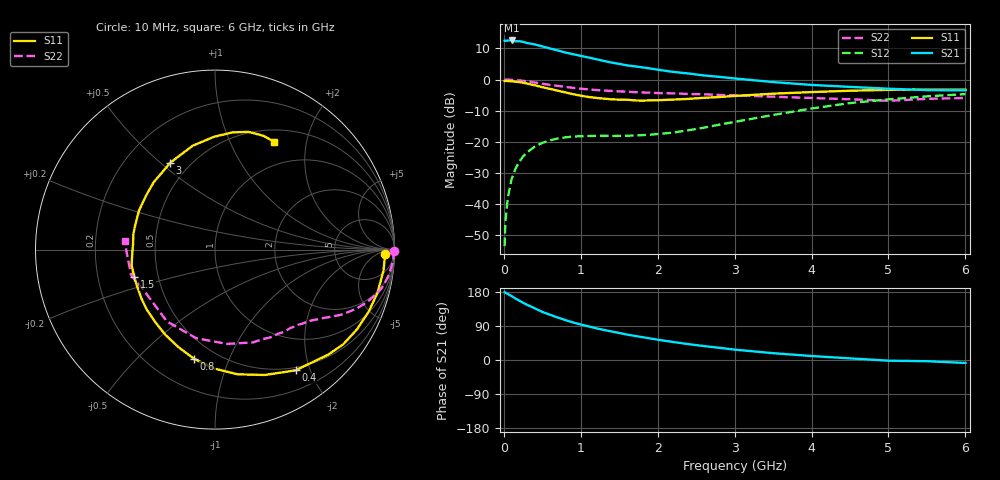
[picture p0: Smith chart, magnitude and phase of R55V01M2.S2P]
! SIEMENS Small Signal Semiconductors
! BFR183
! Si NPN RF Bipolar Junction Transistor in SOT23
! VCE = 5 V  IC = 1.2 mA
! Common Emitter S-Parameters:  May  1996
# GHz  S  MA  R  50
!  f  S11  S21  S12  S22
! GHz  MAG  ANG  MAG  ANG  MAG  ANG  MAG  ANG
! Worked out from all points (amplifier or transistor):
!   36 points, 10 MHz to 6 GHz, reference 50 ohm
!   highest |S21| = 12.5 dB at 100 MHz (marker M1)
!   |S21| within 3 dB of that: start of sweep to 667.1 MHz
!   unconditionally stable (mu >= 1): 1.612 GHz to 2.909 GHz
!   at 250 MHz: K = 0.17, MSG = 18.4 dB, |S12| = -24.7 dB
!   at 1.4 GHz: K = 0.89, MSG = 11.8 dB, |S12| = -18.1 dB
!   at 6 GHz: K = 0.94, MSG = 0.6 dB, |S12| = -4.7 dB
!   S11 on the Smith chart (normalised r, x): 10 MHz: 30, -14; 400 MHz: 0.46, -1.78; 800 MHz: 0.38, -0.75; 1.5 GHz: 0.36, -0.14; 3 GHz: 0.39, +0.54; 6 GHz: 0.65, +1.48
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0.01  0.9473 -1.5  4.218 179.2  0.0021 92.5  0.9986 -0.5
0.02  0.947 -3.0  4.15 177.6  0.0051 94.8  0.9915 -1.0
0.05  0.9461 -7.2  4.236 174.3  0.0123 86.0  0.9958 -2.8
0.1  0.9368 -14.9  4.24 168.8  0.0249 81.0  0.9878 -5.5
0.15  0.9232 -22.1  4.112 162.2  0.0365 77.1  0.9797 -8.2
0.2  0.9078 -29.2  4.121 156.7  0.0477 72.9  0.9668 -10.6
0.25  0.8882 -36.5  4.025 151.1  0.0579 68.5  0.9515 -13.2
0.4  0.8087 -56.3  3.668 136.6  0.0835 58.4  0.8959 -19.1
0.5  0.7519 -68.3  3.403 126.9  0.0958 52.6  0.8545 -22.6
0.7  0.662 -90.6  2.932 112.1  0.1127 43.9  0.7899 -27.4
0.8  0.6194 -100.8  2.711 105.3  0.1176 40.6  0.7597 -29.2
0.9  0.5811 -110.4  2.553 99.0  0.1214 38.2  0.7346 -30.9
1.1  0.5236 -129.4  2.258 88.7  0.1237 35.4  0.6934 -34.0
1.3  0.4924 -146.2  1.988 79.4  0.1249 34.4  0.6645 -36.5
1.5  0.4753 -161.4  1.786 71.4  0.1244 35.2  0.6451 -39.1
1.9  0.4628 169.6  1.505 56.9  0.1294 41.9  0.6131 -44.8
2.2  0.4758 152.9  1.326 47.5  0.14 47.5  0.5996 -49.7
3  0.5442 117.4  1.04 27.4  0.2085 56.8  0.5591 -67.6
3.5  0.5919 102.1  0.91 18.0  0.2695 55.1  0.5294 -83.0
4.5  0.6602 81.6  0.761 4.3  0.4183 42.7  0.4817 -123.8
5.5  0.6891 67.0  0.675 -3.2  0.5361 26.3  0.4886 -163.4
6  0.6854 61.4  0.669 -7.8  0.5831 16.4  0.5058 174.7
